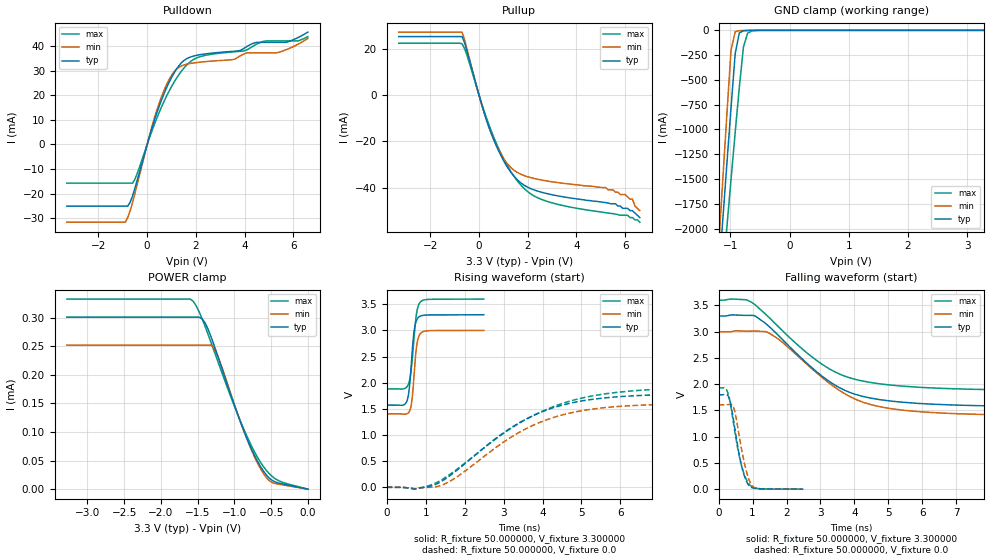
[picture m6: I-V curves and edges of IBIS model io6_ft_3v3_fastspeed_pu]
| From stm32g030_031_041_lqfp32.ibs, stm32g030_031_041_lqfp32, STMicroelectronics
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|   Model io6_ft_3v3_fastspeed_pu
[Model]  io6_ft_3v3_fastspeed_pu
Model_type I/O
Polarity   Non-Inverting
Enable   Active-Low
Vinl =   0.990000V
Vinh =   2.310000V
Vmeas =  1.650000V
Cref =   50.000000pF
Rref =   100.000000M
Vref =   0.0V
C_comp   1.290400pF   1.272500pF   1.305600pF
[Temperature Range]   25.000000   -40.000000   0.125000k
[Pullup Reference]   3.300000V   3.000000V   3.600000V
[Pulldown Reference]   0.0V   0.0V   0.0V
[POWER Clamp Reference]   3.300000V   3.000000V   3.600000V
[GND Clamp Reference]   0.0V   0.0V   0.0V
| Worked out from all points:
|   slope of the pulldown table from 0 to 0.495 V, typ, clamps not added: 31.8 ohm
|   slope of the pullup table from 0 to 0.495 V, typ, clamps not added: 30.4 ohm
|   GND clamp passes 1 mA (typ) near -0.65 V on its own axis
|   rising waveform, R_fixture 50.000000, V_fixture 3.300000: 20-80 % time 114ps typ, 109ps min, 129ps max; typ from 1.57 V to 3.3 V
|   rising waveform, R_fixture 50.000000, V_fixture 0.0: 20-80 % time 2.11ns typ, 2.05ns min, 2.4ns max; typ from 0.002 V to 1.8 V
|   falling waveform, R_fixture 50.000000, V_fixture 3.300000: 20-80 % time 1.89ns typ, 1.91ns min, 1.95ns max; typ from 3.3 V to 1.57 V
|   falling waveform, R_fixture 50.000000, V_fixture 0.0: 20-80 % time 300ps typ, 289ps min, 333ps max; typ from 1.8 V to 0.002 V
[Pulldown]
|Voltage   I(typ)   I(min)   I(max)
-3.3V     -25.03mA   -31.54mA   -15.7mA
-900mV    -25.03mA   -31.54mA   -15.7mA
-700mV    -23.48mA   -26.95mA   -15.7mA
-500mV    -17.69mA   -19.75mA   -14.07mA
100mV     3.479mA    3.853mA    2.862mA
500mV     15.71mA    16.96mA    13.17mA
900mV     25.22mA    26.33mA    21.66mA
1.3V      31.91mA    31.32mA    28.29mA
2.2V      36.48mA    33.43mA    35.69mA
4.1V      39.76mA    37.15mA    38.42mA
5.3V      41.43mA    37.15mA    42.02mA
6.6V      45.6mA     43.04mA    43.74mA
[Pullup]
|Voltage   I(typ)   I(min)   I(max)
-3.3V     25.49mA    27.43mA    22.6mA
-700mV    25.49mA    27.43mA    22.39mA
-500mV    19.3mA     20.21mA    17.46mA
100mV     -3.672mA   -3.825mA   -3.371mA
600mV     -19.12mA   -19.15mA   -18.08mA
1.1V      -30.05mA   -28.8mA    -29.38mA
1.7V      -37.83mA   -34.15mA   -38.73mA
2.8V      -42.64mA   -37.15mA   -46mA
5.2V      -46.5mA    -40mA      -50.9mA
6.3V      -50mA      -45mA      -53mA
6.4V      -51mA      -48mA      -54mA
6.6V      -53mA      -50mA      -55mA
[GND_clamp]
|Voltage   I(typ)   I(min)   I(max)
-3.3V     -9.61A     -9.635A    -9.699A
-1.2V     -2.493A    -2.184A    -2.958A
-1.13V    -1.917A    -1.512A    -2.469A
-1.06V    -1.345A    -845.6mA   -1.983A
-990mV    -779.8mA   -200.2mA   -1.503A
-920mV    -235.5mA   -14.18mA   -1.03A
-850mV    -26.06mA   -3.338mA   -574.2mA
-780mV    -4.499mA   -1.808mA   -166.4mA
-710mV    -1.722mA   -869.6uA   -29.45mA
-640mV    -806.7uA   -283.7uA   -6.281mA
3.28V     0A         0A         0A
[POWER_clamp]
|Voltage   I(typ)   I(min)   I(max)
-3.28V    300.8uA    252uA      332.4uA
-1.6V     300.8uA    252uA      332.4uA
-1.56V    300.8uA    252uA      328.4uA
-1.44V    297.9uA    252uA      298.3uA
-1.36V    280.4uA    252uA      271.4uA
-1.28V    252.9uA    246.9uA    243.1uA
-1.2V     222.5uA    224.3uA    214.5uA
-920mV    118.6uA    118.8uA    119.5uA
-680mV    47.6uA     44.33uA    54.63uA
-560mV    24.08uA    19.48uA    32.08uA
-480mV    14.89uA    11.29uA    21.67uA
0V        0A         0A         0A
[Ramp]
| variable   typ   min   max
dV/dt_r  1.07348/2.09581n   0.96120/2.04204n   1.14413/2.37702n
dV/dt_f  1.02792/1.87135n   0.94800/1.89025n   1.02144/1.93042n
R_load = 50.000000
[Rising Waveform]
R_fixture= 50.000000
V_fixture= 3.300000
V_fixture_min= 3.000000
V_fixture_max= 3.600000
|time   V(typ)   V(min)   V(max)
0s        1.573V     1.405V     1.883V
435.4ps   1.577V     1.401V     1.884V
510.5ps   1.636V     1.404V     1.915V
560.6ps   1.78V      1.429V     1.979V
635.6ps   2.391V     1.601V     2.298V
700.7ps   2.971V     2.119V     2.852V
760.8ps   3.182V     2.656V     3.296V
820.8ps   3.254V     2.878V     3.487V
1.031ns   3.295V     2.993V     3.591V
2.492ns   3.3V       3V         3.6V
[Rising Waveform]
R_fixture= 50.000000
V_fixture= 0.0
V_fixture_min= 0.0
V_fixture_max= 0.0
|time   V(typ)   V(min)   V(max)
0s        1.557mV    1.173mV    2.432mV
780.8ps   -19.42mV   -19.79mV   -27.93mV
1.161ns   31.17mV    3.07mV     53.19mV
1.461ns   141.2mV    57.15mV    168.4mV
3.243ns   1.163V     983.2mV    1.154V
3.844ns   1.401V     1.216V     1.402V
4.585ns   1.588V     1.399V     1.622V
5.305ns   1.686V     1.498V     1.752V
6.346ns   1.751V     1.565V     1.847V
9.97ns    1.797V     1.608V     1.926V
[Falling Waveform]
R_fixture= 50.000000
V_fixture= 3.300000
V_fixture_min= 3.000000
V_fixture_max= 3.600000
|time   V(typ)   V(min)   V(max)
0s        3.3V       3V         3.6V
820.8ps   3.312V     3.011V     3.605V
1.081ns   3.297V     3.013V     3.509V
1.441ns   3.125V     2.989V     3.298V
2.903ns   2.228V     2.208V     2.445V
3.443ns   1.977V     1.933V     2.229V
3.984ns   1.817V     1.728V     2.099V
4.685ns   1.713V     1.58V      2.013V
5.866ns   1.635V     1.479V     1.944V
9.97ns    1.573V     1.405V     1.883V
[Falling Waveform]
R_fixture= 50.000000
V_fixture= 0.0
V_fixture_min= 0.0
V_fixture_max= 0.0
|time   V(typ)   V(min)   V(max)
0s        1.797V     1.608V     1.926V
250.2ps   1.798V     1.61V      1.871V
340.3ps   1.67V      1.618V     1.647V
435.4ps   1.332V     1.569V     1.272V
575.6ps   767.8mV    1.136V     735.2mV
685.7ps   420.9mV    727.2mV    423.3mV
800.8ps   179.3mV    382mV      208.1mV
925.9ps   51.67mV    132.2mV    75.76mV
1.181ns   9.789mV    12.46mV    11.36mV
2.492ns   1.557mV    1.173mV    2.432mV
